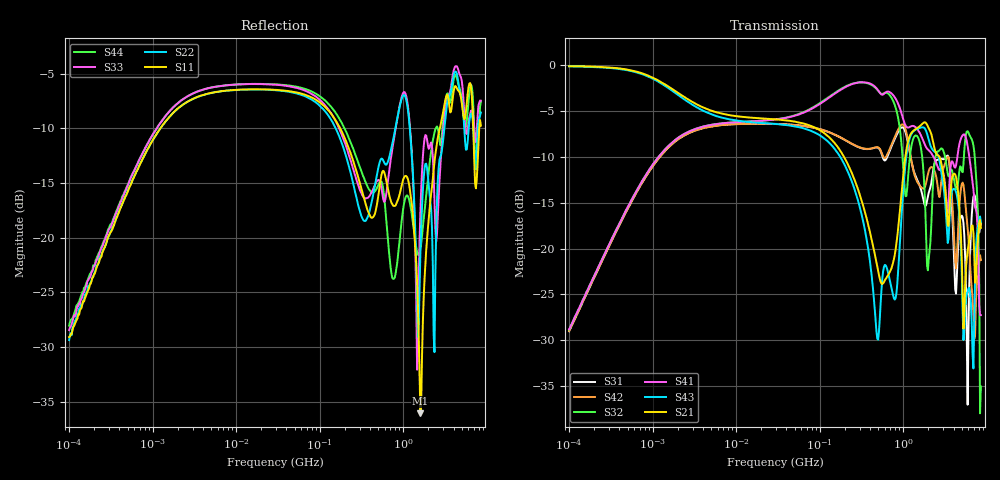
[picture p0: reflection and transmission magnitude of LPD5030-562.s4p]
# MHz S MA R 50
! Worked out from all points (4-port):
!   498 points, 100 kHz to 8.5 GHz, reference 50 ohm
!   strongest paths, dB at 100 kHz, 1.698 MHz, 29.49 MHz, 500.7 MHz, 8.5 GHz:
!     S21: -0.1, -2.5, -5.9, -22.4, -17.7
!     S43: -0.1, -2.7, -6.4, -29.9, -17.1
!     S41: -28.8, -8.5, -5.9, -2.7, -27.3
!     S32: -28.8, -8.4, -5.9, -2.8, -35.1
!     S42: -29.0, -8.6, -6.4, -8.9, -21.2
!     S31: -29.0, -8.6, -6.4, -9.0, -17.3
!   lowest |S11| = -36.1 dB at 1.605 GHz (marker M1), VSWR 1.03, Z = 51.4 - j0.807 ohm
!   |S11| at or under -10 dB: start of sweep to 1.238 MHz; 175.4 MHz to 2.744 GHz (2.569 GHz wide, 176 % of centre); 6.888 GHz to 8.121 GHz (1.233 GHz wide, 16.4 % of centre)
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0.1  0.03504 82.6  0.9909 -2.1  0.03541 -94.9  0.03633 85.4
     0.9909 -2.1  0.03398 82.6  0.03612 85.4  0.03556 -94.5
     0.03541 -94.9  0.03612 85.4  0.03774 80.0  0.9888 -2.3
     0.03633 85.4  0.03556 -94.5  0.9888 -2.3  0.03948 83.0
38.78723  0.4694 -14.6  0.5023 -20.3  0.4774 160.2  0.5168 4.6
          0.5023 -20.3  0.4666 -14.2  0.5185 4.3  0.4771 160.4
          0.4774 160.2  0.5185 4.3  0.4945 -13.8  0.4734 -21.1
          0.5168 4.6  0.4771 160.4  0.4734 -21.1  0.4979 -14.1
489.3566  0.1449 -78.3  0.07979 179.9  0.3568 -2.8  0.7421 -82.0
          0.07979 179.9  0.1976 -43.7  0.7369 -89.7  0.358 -1.7
          0.3568 -2.8  0.7369 -89.7  0.1816 -61.1  0.03222 127.8
          0.7421 -82.0  0.358 -1.7  0.03222 127.8  0.17 -102.1
1604.647  0.0157 -30.0  0.4698 177.2  0.2152 141.5  0.4216 116.4
          0.4698 177.2  0.08502 178.8  0.3675 100.4  0.2186 145.9
          0.2152 141.5  0.3675 100.4  0.1319 -160.7  0.4576 170.6
          0.4216 116.4  0.2186 145.9  0.4576 170.6  0.089 -55.6
3111.8  0.4045 5.6  0.2311 -78.8  0.3091 -66.4  0.2391 -75.1
        0.2311 -78.8  0.3189 15.8  0.3279 -59.9  0.2852 -58.9
        0.3091 -66.4  0.3279 -59.9  0.3524 9.9  0.198 -90.3
        0.2391 -75.1  0.2852 -58.9  0.198 -90.3  0.3879 6.2
6764.496  0.3801 162.9  0.1339 -145.4  0.1765 -117.8  0.2296 145.1
          0.1339 -145.4  0.3474 -152.9  0.3832 151.0  0.05305 150.0
          0.1765 -117.8  0.3832 151.0  0.3786 -146.0  0.0264 132.2
          0.2296 145.1  0.05305 150.0  0.0264 132.2  0.4566 -157.4
8500  0.3248 -42.6  0.1298 -2.5  0.1364 -2.9  0.04337 -74.9
      0.1298 -2.5  0.3729 -37.2  0.01768 -19.3  0.08668 -15.3
      0.1364 -2.9  0.01768 -19.3  0.4222 -38.1  0.1399 23.8
      0.04337 -74.9  0.08668 -15.3  0.1399 23.8  0.4178 -34.7
